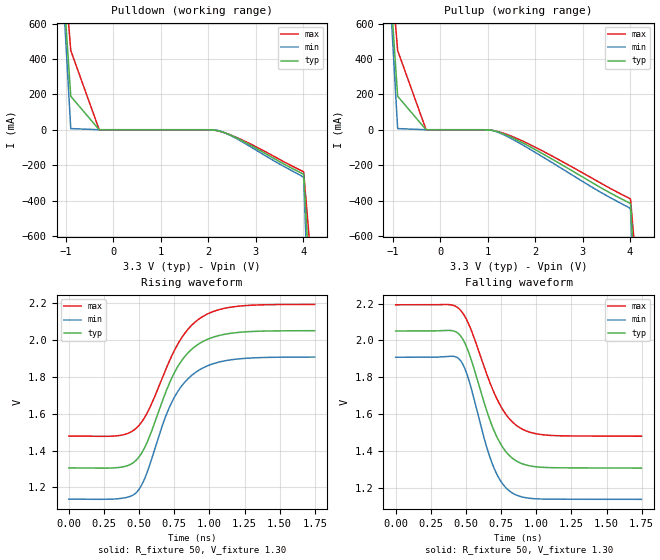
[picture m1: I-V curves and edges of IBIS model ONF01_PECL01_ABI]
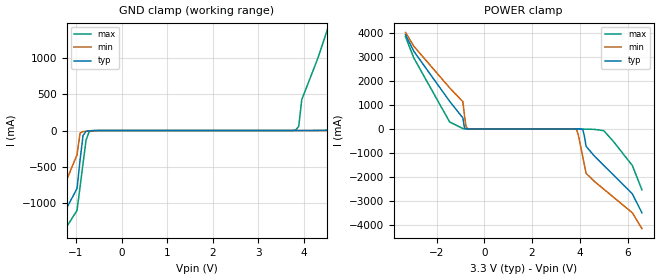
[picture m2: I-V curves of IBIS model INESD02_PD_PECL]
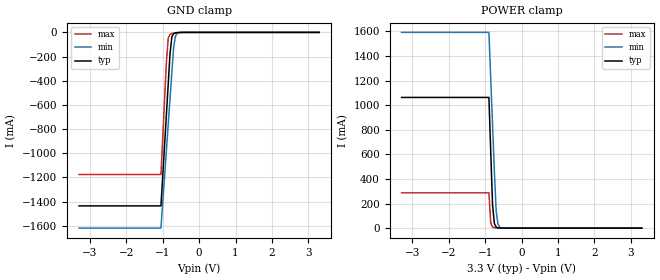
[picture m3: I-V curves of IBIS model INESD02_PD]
|   This file is an IBIS representation of the   |
|   Integrated Devices Technology, Inc.   |
|   ICS843004-125   |
|   FEMTOCLOCKS CRYSTAL-TO-3.3V LVPECL FREQUENCY SYNTHESIZER   |
[IBIS Ver]   4.1
[File name]   843004_125_3v3.ibs
[File Rev]   1.0
[Date]   1 Jun 2010
[Source]   Originated at Integrated Device Technology, Inc.
[Disclaimer]
IDT hereby grants the user of this IBIS model a non-exclusive,
nontransferable license to use this IBIS model under the following terms.
Before using this IBIS model, the user should read this license.
If the user does not accept these terms,  the IBIS model should be
returned to IDT within 30 days.
   The user is granted this license only to use the IBIS model and
is not granted rights to sell, load, rent, lease or license the IBIS
model in whole or in part, or in modified form to anyone other than
user. User may modify the IBIS model to suit its specific
applications but rights to derivative works and such modifications
shall belong to IDT.
   This IBIS model is provided on an "AS IS" basis and IDT makes
absolutely no warranty with respect to the information contained
herein. IDT DISCLAIMS AND CUSTOMER WAIVES ALL WARRANTIES, EXPRESS
OR IMPLIED, INCLUDING WARRANTIES OF MERCHANTABILITY OR FITNESS FOR
A PARTICULAR PURPOSE. The entire risk as to quality and performance
is with the Customer. ACCORDINGLY, IN NO EVENT SHALL THE COMPANY BE
LIABLE FOR ANY DAMAGES, WHETHER IN CONTRACT OR TORT,INCLUDING ANY
LOST PROFITS OR OTHER INCIDENTAL, CONSEQUENTIAL, EXEMPLARY, OR
PUNITIVE DAMAGES ARISING OUT OF THE USE OR APPLICATION OF THE IBIS
model provided in this package. Further, IDT reserves the right to
make changes without notice to any product herein to improve
reliability, function, or design. IDT does not convey any license
under patent rights or any other intellectual property rights,
including those of third parties.
   IDT is not obligated to provide maintenance or support
for the licensed IBIS model.
[Copyright]   Copyright 2004 byIntegrated Devices Technology, Inc.
[Component]   ICS843004G-125
[Manufacturer] Integrated Device Technology, Inc.
[Package]
|TSSOP 24 Lead
|   typ   min   max
R_pkg   60.65m   52.4m   68.9m
L_pkg   1.989nH   1.431nH   2.547nH
C_pkg   0.314pF   0.254pF   0.374pF
[Pin]   signal_name   model_name   R_pin   L_pin   C_pin
1   nQ1   ONF01_PECL01_ABI   68.9m   2.547n   0.374p
2   Q1   ONF01_PECL01_ABI   65.6m   2.323n   0.350p
3   VCCO   POWER   62.3m   2.100n   0.326p
4   Q0   ONF01_PECL01_ABI   59.0m   1.877n   0.302p
5   nQ0   ONF01_PECL01_ABI   55.7m   1.654n   0.278p
6   MR   INESD02_PD_PECL   52.4m   1.431n   0.254p
7   nPLL_SEL   INESD02_PD   52.4m   1.431n   0.254p
8   NC   NC   55.7m   1.654n   0.278p
9   VCCA   POWER   59.0m   1.877n   0.302p
10  NC   NC   62.3m   2.100n   0.326p
11  VCC   POWER   65.6m   2.323n   0.350p
12  NC   NC   68.9m   2.547n   0.374p
13  XTAL_OUT   NC   68.9m   2.547n   0.374p
14  XTAL_IN   NC   65.6m   2.323n   0.350p
15  VEE   GND   62.3m   2.100n   0.326p
16  REF_CLK   INESD04_PD_PECL   59.0m   1.877n   0.302p
17  nXTAL_SEL   INESD02_PD   55.7m   1.654n   0.278p
18  VCC   POWER   52.4m   1.431n   0.254p
19  VEE   GND   52.4m   1.431n   0.254p
20  nQ3   ONF01_PECL01_ABI   55.7m   1.654n   0.278p
21  Q3   ONF01_PECL01_ABI   59.0m   1.877n   0.302p
22  VCCO   POWER   62.3m   2.100n   0.326p
23  Q2   ONF01_PECL01_ABI   65.6m   2.323n   0.350p
24  nQ2   ONF01_PECL01_ABI   68.9m   2.547n   0.374p
[Diff Pin]  inv_pin  vdiff tdelay_typ tdelay_min  tdelay_max
2   1   NA   0   0   0
21   20   NA   0   0   0
23   24   NA   0   0   0
4   5   NA   0   0   0
| Models and submodels in the file (4): ONF01_PECL01_ABI (Output_ECL), INESD02_PD_PECL (Input), INESD02_PD (Input), INESD04_PD_PECL (Input)
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[Model]   ONF01_PECL01_ABI
Model_type   Output_ECL
Polarity   Non-Inverting
|   typ   min   max
C_comp   2pF   1.5pF   2.5pF
Vmeas = 1.62V
Rref = 50
Cref = 0
Vref = 1.3V
|   typ   min   max
[Voltage range]   3.3V   3.135V   3.465V
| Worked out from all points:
|   rising waveform, R_fixture 50, V_fixture 1.30: 20-80 % time 253ps typ, 244ps min, 269ps max; typ from 1.31 V to 2.05 V
|   falling waveform, R_fixture 50, V_fixture 1.30: 20-80 % time 199ps typ, 176ps min, 223ps max; typ from 2.05 V to 1.31 V
[Pulldown]
|Voltage   I (typ)   I (min)   I (max)
-3.3V     9.786A     12.03A     8.45A
-1.5V     2.58A      2.839A     2.441A
-900mV    189.2mA    6.554mA    448mA
-300mV    38.6nA     139.1pA    1.11uA
1.978V    -80.11uA   -13.25uA   -238.1uA
2.126V    -1.925mA   -870.5uA   -2.993mA
2.274V    -10.73mA   -9.534mA   -11.63mA
2.471V    -31.01mA   -32.89mA   -29.75mA
2.817V    -76.79mA   -84.38mA   -70.9mA
4.01V     -252.1mA   -270.1mA   -237.9mA
4.528V    -2.68A     -3.925A    -1.887A
6.6V      -15.69A    -20.55A    -12.73A
[Pullup]
|Voltage   I (typ)   I (min)   I (max)
-3.3V     9.786A     12.03A     8.45A
-1.5V     2.58A      2.839A     2.441A
-900mV    189.2mA    6.554mA    448mA
-300mV    38.6nA     139.1pA    1.11uA
1.041V    -1.682mA   -1.459mA   -1.692mA
1.288V    -18.79mA   -22.48mA   -15.95mA
1.682V    -66.58mA   -77.82mA   -57.47mA
2.274V    -153.4mA   -172.3mA   -136.7mA
3.26V     -308.2mA   -334.6mA   -283.1mA
4.01V     -417.2mA   -447.3mA   -390.7mA
4.528V    -2.844A    -4.101A    -2.04A
6.6V      -15.79A    -20.6A     -12.84A
[Ramp]
|   typ   min   max
dV/dt_r   0.597/0.406n   0.618/0.395n   0.573/0.427n
dV/dt_f   0.598/0.304n   0.622/0.269n   0.572/0.341n
R_load =   50.0000
[Rising Waveform]
R_fixture = 50
V_fixture = 1.30   | VCC_typ - 2V
V_fixture_max = 1.465   | VCC_max - 2V
V_fixture_min = 1.135   | VCC_min - 2V
C_fixture = 0.0p
| Time   typ   min   max
0s        1.306V     1.136V     1.479V
348.6ps   1.308V     1.138V     1.481V
480ps     1.348V     1.172V     1.522V
546.5ps   1.427V     1.261V     1.589V
672.7ps   1.684V     1.553V     1.81V
741ps     1.808V     1.676V     1.929V
828.6ps   1.914V     1.775V     2.041V
933.7ps   1.984V     1.841V     2.119V
1.184ns   2.04V      1.896V     2.183V
1.748ns   2.051V     1.908V     2.194V
[Falling Waveform]
R_fixture = 50
V_fixture = 1.30   | VCC_typ - 2V
V_fixture_max = 1.465   | VCC_max - 2V
V_fixture_min = 1.135   | VCC_min - 2V
C_fixture = 0.0p
| Time   typ   min   max
0s        2.052V     1.909V     2.194V
380.1ps   2.055V     1.914V     2.195V
457.2ps   2.029V     1.894V     2.168V
516.8ps   1.94V      1.794V     2.093V
634.1ps   1.65V      1.454V     1.846V
691.9ps   1.524V     1.32V      1.73V
756.8ps   1.424V     1.224V     1.63V
833.8ps   1.358V     1.169V     1.554V
1.053ns   1.31V      1.138V     1.487V
1.748ns   1.306V     1.136V     1.479V
[Model]   INESD02_PD_PECL
Model_type  Input
Polarity   Non-Inverting
Vinl = 0.8V
Vinh = 2.0V
|   typ   min   max
C_comp   2pF   1.5pF   2.5pF
|   typ   min   max
[Voltage range]  3.3V   3.135V   3.465V
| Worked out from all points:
|   GND clamp passes 1 mA (typ) near -0.59 V on its own axis
|   POWER clamp passes 1 mA (typ) near -0.70 V on its own axis
[GND_clamp]
-3.3V     -3.894A    -4.294A    -3.674A
-1.6V     -1.569A    -1.322A    -1.74A
-974.8mV  -794.1mA   -331.5mA   -1.096A
-843.4mV  -68.33mA   -15.34mA   -452.9mA
-646.5mV  -1.912mA   -4.151mA   -2.665mA
3.818V    89.38uA    70.49uA    7.198mA
3.95V     342.2uA    75.94uA    423.8mA
4.6V      7.437mA    165.5uA    1.553A
4.9V      78.32mA    440.9uA    2.118A
5.5V      1.293A     2.769mA    3.249A
6.25V     2.651A     112.4mA    4.38A
6.6V      3.331A     896.1mA    4.946A
[POWER_clamp]
-3.3V     3.923A     4.017A     3.838A
-2.95V    3.23A      3.44A      2.951A
-1.45V    1.149A     1.709A     289.6mA
-896.9mV  456.5mA    1.133A     15.4mA
-762.9mV  4.223mA    91.07mA    1.486mA
-695.9mV  792.2uA    10.73mA    555.6uA
3.861V    -556.7uA   -26.14mA   -39.45uA
4.129V    -41.85mA   -1.19A     -4.904mA
4.263V    -724.2mA   -1.847A    -12.04mA
5V        -1.514A    -2.505A    -71.38mA
6.2V      -2.701A    -3.492A    -1.525A
6.6V      -3.492A    -4.151A    -2.536A
[Model]   INESD02_PD
Model_type   Input
Polarity   Non-Inverting
Vinl = 0.80V
Vinh = 2.0V
|   typ   min   max
C_comp   2pF   1.5pF   2.5pF
|   typ   min   max
[Voltage range]  3.3V   3.135V   3.465V
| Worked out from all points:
|   GND clamp passes 1 mA (typ) near -0.56 V on its own axis
|   POWER clamp passes 1 mA (typ) near -0.61 V on its own axis
[GND_clamp]
|Voltage   I(typ)   I(min)   I(max)
-3.3V     -1.436A    -1.62A     -1.176A
-1.05V    -1.436A    -1.62A     -1.176A
-900mV    -678.5mA   -975.1mA   -244mA
-850mV    -426.1mA   -760.1mA   -46.85mA
-800mV    -173.9mA   -545.4mA   -16.11mA
-750mV    -36.96mA   -330.7mA   -9.916mA
-700mV    -9.696mA   -120.2mA   -7.056mA
-650mV    -3.545mA   -29.7mA    -4.857mA
-600mV    -1.629mA   -7.52mA    -3.049mA
-400mV    -52.81uA   -52.52uA   -108.7uA
3.3V      71.13uA    77.43uA    62.11uA
[POWER_clamp]
|Voltage   I(typ)   I(min)   I(max)
-3.3V     1.063A     1.593A     287.3mA
-900mV    1.063A     1.593A     287.3mA
-850mV    620.5mA    1.215A     41.84mA
-800mV    191.6mA    837.5mA    8.757mA
-750mV    37.76mA    460.2mA    3.328mA
-700mV    8.104mA    133.8mA    1.728mA
-650mV    2.076mA    32.66mA    905.3uA
-600mV    678.1uA    8.083mA    443.8uA
-450mV    104.2uA    213.3uA    89.09uA
3.3V      -3.041nA   -3.986uA   0A
